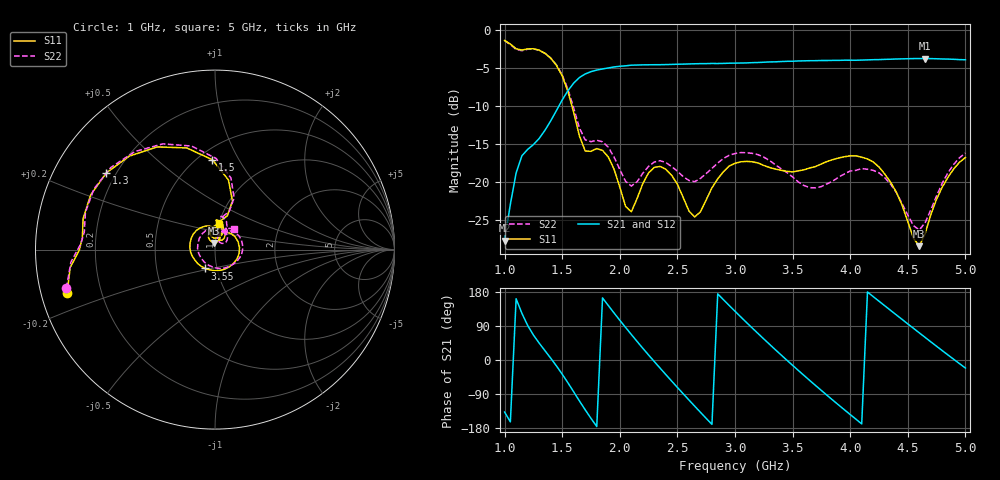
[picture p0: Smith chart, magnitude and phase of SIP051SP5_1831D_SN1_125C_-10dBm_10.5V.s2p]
# GHz  S  dB  R  50
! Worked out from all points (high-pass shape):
!   81 points, 1 GHz to 5 GHz, reference 50 ohm
!   highest |S21| = -3.72 dB at 4.65 GHz (marker M1); lowest = -27.7 dB at 1 GHz (marker M2)
!   |S21| within 3 dB of the highest: 1.616 GHz to end of sweep
!   lowest |S11| = -28.5 dB at 4.6 GHz (marker M3), VSWR 1.08, Z = 49.5 + j3.72 ohm
!   |S11| at or under -10 dB: 1.585 GHz to end of sweep
!   |S22| runs from -26.3 to -1.4 dB; largest |S21 - S12| = 0.0026
!   S11 on the Smith chart (normalised r, x): 1 GHz: 0.08, -0.14; 1.3 GHz: 0.16, +0.31; 1.5 GHz: 0.59, +0.78; 3.55 GHz: 0.88, -0.19; 5 GHz: 1.01, +0.29
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1  -1.33 -163.7  -27.73 -137.3  -27.77 -137.2  -1.36 -165.4
1.15  -2.59 174.9  -16.55 123.2  -16.55 123.4  -2.68 172.3
1.3  -2.60 144.7  -14.26 44.6  -14.25 44.7  -2.63 141.7
1.5  -6.00 91.7  -9.19 -37.4  -9.18 -37.4  -5.88 89.3
1.7  -15.91 79.9  -5.75 -131.6  -5.74 -131.6  -14.45 76.6
1.85  -15.83 81.2  -5.09 163.8  -5.09 163.8  -14.70 74.6
2.05  -23.22 74.3  -4.67 86.0  -4.67 86.1  -19.91 66.4
2.2  -20.20 105.9  -4.55 30.9  -4.55 31.0  -18.84 84.9
2.35  -17.95 81.3  -4.53 -21.5  -4.51 -21.6  -17.19 69.9
2.6  -23.82 53.9  -4.43 -105.5  -4.42 -105.4  -19.80 53.7
2.8  -20.78 74.0  -4.37 -169.8  -4.35 -169.8  -18.21 55.7
3  -17.54 31.6  -4.32 128.6  -4.31 128.7  -16.25 29.1
3.25  -17.82 -36.7  -4.20 55.5  -4.20 55.6  -16.73 -17.0
3.4  -18.46 -79.0  -4.11 13.4  -4.10 13.3  -18.26 -50.8
3.55  -18.53 -117.8  -4.03 -27.6  -4.03 -27.6  -20.00 -92.9
3.7  -17.96 -152.8  -4.00 -67.5  -3.99 -67.4  -20.78 -148.0
3.85  -17.04 175.4  -3.96 -106.2  -3.95 -106.2  -19.87 159.9
4.05  -16.56 133.6  -3.94 -156.2  -3.93 -156.2  -18.47 103.5
4.35  -20.02 77.3  -3.80 131.1  -3.81 131.2  -20.28 44.1
4.6  -28.47 95.5  -3.72 71.5  -3.71 71.5  -26.33 57.4
4.65  -26.82 111.5  -3.72 59.7  -3.73 59.6  -25.39 70.5
5  -16.78 80.1  -3.88 -21.2  -3.88 -21.3  -16.19 47.0
